| IBIS file was generated by Viper version: 2023.04.24
[IBIS Ver]   5.0
[Comment Char]   |_char
[File Name]   imxrt1180_c0_bga196_consmr.ibs
[File Rev]   1
[Date]   Thu Jan 23 17:55:28 2025
[Source]   NXP Viper 2023.04.24
[Notes]
[Disclaimer] IMPORTANT NOTICE
  This information is provided on an AS IS basis and without warranty.
  IN NO EVENT SHALL NXP BE LIABLE FOR INCIDENTAL OR CONSEQUENTIAL
  DAMAGES ARISING FROM USE OF THIS INFORMATION. THIS DISCLAIMER OF
  WARRANTY EXTENDS TO THE USER OF THE INFORMATION, AND TO THEIR CUSTOMERS
  OR USERS OF PRODUCTS  AND IS IN LIEU OF ALL WARRANTIES WHETHER EXPRESS,
  IMPLIED, OR STATUTORY, INCLUDING IMPLIED WARRANTIES OF MERCHANTABILITY
  OR FITNESS FOR PARTICULAR PURPOSE.
  NXP does not represent or warrant that the information furnished
  hereunder is free of infringement of any third party patents,
  copyrights, trade secrets, or other intellectual property rights.
  NXP does not represent or warrant that the information is free of
  defect, or that it meets any particular standard, requirements or need
  of the user of the infomation or their customers.
  NXP reserves the right to change the information in this file
  without notice.
   http://www.nxp.com
[Copyright]   (C) Copyright NXP 2004 - 2025, All Rights Reserved.
|   BGA196
[Component]   imxrt1180_bga196
[Manufacturer]   NXP
[Package]
| variable   typ   min   max
R_pkg   0.26256   0.042833   0.47223
L_pkg   3.535e-09   7.477e-10   7.758e-09
C_pkg   7.130e-13   4.458e-13   2.812e-12
[Pin] signal_name   model_name   R_pin   L_pin   C_pin
A1   VSS   GND   NA   NA   NA
A2   GPIO_EMC_B1_09   STGPIO   0.35642   4.603e-09 7.554e-13
A3   GPIO_AON_20   FSGPIO   0.21508   3.819e-09 5.831e-13
A4   GPIO_AON_19   FSGPIO   0.22197   4.065e-09 5.641e-13
A5   GPIO_AON_25   FSGPIO   0.3641   5.392e-09 5.514e-13
A6   GPIO_AON_24   FSGPIO   0.37702   4.913e-09 5.483e-13
A7   GPIO_AON_08   FSGPIO   0.37054   5.150e-09 5.122e-13
A8   GPIO_AON_12   FSGPIO   0.36547   5.045e-09 5.397e-13
A9   GPIO_AON_13   FSGPIO   0.39395   5.434e-09 5.821e-13
A10   GPIO_AON_01   FSGPIO   0.30629   5.038e-09 5.883e-13
A11   GPIO_AON_00   FSGPIO   0.29989   5.266e-09 6.848e-13
A12   GPIO_B2_07   STGPIO   0.47215   7.758e-09 9.398e-13
A13   GPIO_B2_08   STGPIO   0.47223   7.123e-09 9.633e-13
A14   VSS   GND   NA   NA   NA
B1   GPIO_EMC_B1_17   STGPIO   0.36515   4.326e-09 6.932e-13
B2   GPIO_EMC_B1_18   STGPIO   0.32419   3.726e-09 7.722e-13
B3   GPIO_AON_27   FSGPIO   0.26934   3.420e-09 5.231e-13
B4   GPIO_AON_26   FSGPIO   0.32404   4.795e-09 5.692e-13
B5   GPIO_AON_18   FSGPIO   0.24149   4.062e-09 5.595e-13
B6   GPIO_AON_23   FSGPIO   0.37852   5.044e-09 5.594e-13
B7   GPIO_AON_22   FSGPIO   0.39361   5.361e-09 5.709e-13
B8   GPIO_AON_15   FSGPIO   0.38558   5.824e-09 5.776e-13
B9   GPIO_AON_14   FSGPIO   0.40673   5.776e-09 6.039e-13
B10   GPIO_AON_11   FSGPIO   0.4088   6.162e-09 6.679e-13
B11   GPIO_AON_10   FSGPIO   0.40617   6.314e-09 6.924e-13
B12   GPIO_AON_09   FSGPIO   0.41769   6.788e-09 7.177e-13
B13   GPIO_B2_13   STGPIO   0.42759   6.730e-09 1.022e-12
B14   GPIO_B2_12   STGPIO   0.45182   7.389e-09 1.035e-12
C1   GPIO_EMC_B1_23   STGPIO   0.37543   4.204e-09 6.553e-13
C2   GPIO_EMC_B1_10   STGPIO   0.33639   3.642e-09 6.362e-13
C3   GPIO_EMC_B1_29   STGPIO   0.15709   2.341e-09 5.594e-13
C4   GPIO_AON_21   FSGPIO   0.10056   1.277e-09 6.902e-13
C5   GPIO_AON_17   FSGPIO   0.15303   1.931e-09 4.458e-13
C6   GPIO_AON_07   FSGPIO   0.15321   2.035e-09 4.695e-13
C7   GPIO_AON_06   FSGPIO   0.20767   2.944e-09 5.496e-13
C8   GPIO_AON_05   FSGPIO   0.26873   4.297e-09 6.302e-13
C9   GPIO_AON_02   FSGPIO   0.26227   4.486e-09 6.748e-13
C10   GPIO_B2_03   STGPIO   0.227   3.500e-09 9.260e-13
C11   GPIO_B2_05   STGPIO   0.28762   4.737e-09 9.986e-13
C12   GPIO_B2_00   STGPIO   0.32395   5.538e-09 1.004e-12
C13   GPIO_B2_10   STGPIO   0.41221   6.592e-09 8.958e-13
C14   GPIO_B2_11   STGPIO   0.44381   7.319e-09 9.732e-13
D1   GPIO_EMC_B1_15   STGPIO   0.36793   4.383e-09 6.235e-13
D2   GPIO_EMC_B1_20   STGPIO   0.34082   4.036e-09 6.104e-13
D3   GPIO_EMC_B1_11   STGPIO   0.34343   4.504e-09 6.504e-13
D4   VSS   GND   NA   NA   NA
D5   GPIO_EMC_B1_28   STGPIO   0.1112   1.432e-09 8.313e-13
D6   GPIO_AON_16   FSGPIO   0.09263   1.103e-09 5.826e-13
D7   NVCC_AON   POWER   NA   NA   NA
D8   GPIO_AON_03   FSGPIO   0.1963   3.001e-09 6.671e-13
D9   GPIO_B2_01   STGPIO   0.21713   2.881e-09 1.080e-12
D10   GPIO_B2_09   STGPIO   0.32026   5.525e-09 1.084e-12
D11   GPIO_B2_02   STGPIO   0.25143   3.934e-09 9.558e-13
D12   VSS   GND   NA   NA   NA
D13   USB1_DP   NC   0.2651   2.959e-09 6.312e-13
D14   USB1_DN   NC   0.25268   3.083e-09 6.395e-13
E1   GPIO_EMC_B1_05   STGPIO   0.23832   3.373e-09 6.272e-13
E2   GPIO_EMC_B1_16   STGPIO   0.31197   3.749e-09 6.419e-13
E3   GPIO_EMC_B1_13   STGPIO   0.1608   1.956e-09 6.369e-13
E4   GPIO_EMC_B1_19   STGPIO   0.098234  1.236e-09 7.015e-13
E5   GPIO_EMC_B1_12   STGPIO   0.098212  1.265e-09 6.870e-13
E6   GPIO_EMC_B1_03   STGPIO   0.13042   1.980e-09 8.047e-13
E7   GPIO_AON_04   FSGPIO   0.18605   2.492e-09 7.514e-13
E8   GPIO_B2_06   STGPIO   0.19268   2.582e-09 1.079e-12
E9   GPIO_B2_04   STGPIO   0.19249   2.700e-09 1.077e-12
E10   GPIO_SD_B1_03   STGPIO   0.24696   2.917e-09 9.185e-13
E11   VDD_USB_3P3   POWER   NA   NA   NA
E12   VDD_USB_1P8   POWER   NA   NA   NA
E13   GPIO_SD_B2_08   STGPIO   0.29716   3.541e-09 5.748e-13
E14   USB1_VBUS   POWER   0.18698   2.479e-09 6.560e-13
F1   GPIO_EMC_B1_31   STGPIO   0.34863   3.980e-09 5.917e-13
F2   GPIO_EMC_B1_30   STGPIO   0.31813   3.449e-09 5.603e-13
F3   GPIO_EMC_B1_08   STGPIO   0.17187   2.258e-09 6.398e-13
F4   GPIO_EMC_B1_14   STGPIO   0.15057   1.843e-09 6.464e-13
F5   GPIO_EMC_B1_01   STGPIO   0.11596   1.557e-09 7.297e-13
F6   NVCC_EMC1   POWER   NA   NA   NA
F7   VSS   GND   NA   NA   NA
F8   VSS   GND   NA   NA   NA
F9   VDD_SOC   POWER   NA   NA   NA
F10   GPIO_SD_B1_02   STGPIO   0.12357   1.900e-09 9.082e-13
F11   GPIO_SD_B2_03   STGPIO   0.21146   2.290e-09 6.433e-13
F12   GPIO_SD_B2_05   STGPIO   0.20101   2.322e-09 6.367e-13
F13   GPIO_SD_B2_11   STGPIO   0.29205   3.573e-09 5.872e-13
F14   GPIO_SD_B2_07   STGPIO   0.32121   4.153e-09 5.878e-13
G1   GPIO_EMC_B1_32   STGPIO   0.33057   3.828e-09 5.129e-13
G2   GPIO_EMC_B1_02   STGPIO   0.25413   3.884e-09 6.301e-13
G3   GPIO_EMC_B1_00   STGPIO   0.1527   1.898e-09 5.702e-13
G4   VSS   GND   NA   NA   NA
G5   GPIO_EMC_B1_27   STGPIO   0.19887   2.581e-09 7.781e-13
G6   NVCC_EMC1   POWER   NA   NA   NA
G7   VSS   GND   NA   NA   NA
G8   VDD_SOC   POWER   NA   NA   NA
G9   VDD_SOC   POWER   NA   NA   NA
G10   NVCC_SD2   POWER   NA   NA   NA
G11   VSS   GND   NA   NA   NA
G12   GPIO_SD_B2_04   STGPIO   0.20136   2.455e-09 5.936e-13
G13   GPIO_SD_B2_06   STGPIO   0.29033   3.676e-09 6.032e-13
G14   GPIO_SD_B2_09   STGPIO   0.31752   4.313e-09 5.550e-13
H1   GPIO_EMC_B1_33   STGPIO   0.34284   3.995e-09 5.590e-13
H2   GPIO_EMC_B1_35   STGPIO   0.31001   3.663e-09 5.512e-13
H3   GPIO_EMC_B1_34   STGPIO   0.31772   4.079e-09 5.714e-13
H4   GPIO_EMC_B1_06   STGPIO   0.16355   2.111e-09 7.119e-13
H5   GPIO_EMC_B1_04   STGPIO   0.1908   2.611e-09 7.576e-13
H6   GPIO_EMC_B1_21   STGPIO   0.18972   2.544e-09 7.609e-13
H7   VSS   GND   NA   NA   NA
H8   VDD_SOC   POWER   NA   NA   NA
H9   VDD_SOC   POWER   NA   NA   NA
H10   NVCC_SD2   POWER   NA   NA   NA
H11   GPIO_SD_B2_01   STGPIO   0.22799   3.317e-09 6.041e-13
H12   VDDA_ADC_3P3   POWER   NA   NA   NA
H13   GPIO_SD_B2_10   STGPIO   0.30632   3.978e-09 5.504e-13
H14   GPIO_SD_B2_02   STGPIO   0.33652   3.878e-09 5.752e-13
J1   GPIO_EMC_B1_37   STGPIO   0.32323   3.485e-09 5.526e-13
J2   GPIO_EMC_B1_36   STGPIO   0.37907   4.542e-09 6.302e-13
J3   GPIO_EMC_B1_24   STGPIO   0.15666   1.982e-09 5.863e-13
J4   GPIO_EMC_B1_22   STGPIO   0.17751   2.520e-09 6.260e-13
J5   GPIO_EMC_B1_07   STGPIO   0.10368   1.310e-09 6.824e-13
J6   GPIO_EMC_B1_25   STGPIO   0.18635   2.288e-09 8.252e-13
J7   GPIO_EMC_B1_26   STGPIO   0.2608   3.161e-09 8.827e-13
J8   GPIO_EMC_B2_12   STGPIO   0.19517   3.479e-09 8.111e-13
J9   GPIO_BBSM_05   NC   0.1742   2.674e-09 8.790e-13
J10   VDDA_1P8_IN   POWER   NA   NA   NA
J11   GPIO_SD_B2_00   STGPIO   0.2566   3.930e-09 6.694e-13
J12   DAC_OUT   NC   0.10066   1.340e-09 6.040e-13
J13   VDDA_ADC_1P8   POWER   NA   NA   NA
J14   ADC_VREFH   NC   0.17697   2.908e-09 6.279e-13
K1   GPIO_EMC_B1_39   STGPIO   0.33974   4.342e-09 5.830e-13
K2   GPIO_EMC_B1_38   STGPIO   0.35126   4.532e-09 6.394e-13
K3   DCDC_PSWITCH   NC   0.24821   2.705e-09 6.677e-13
K4   VSS   GND   NA   NA   NA
K5   DCDC_1P8   POWER   0.11971   1.732e-09 9.329e-13
K6   GPIO_EMC_B2_02   STGPIO   0.16558   2.154e-09 6.342e-13
K7   NVCC_EMC2   POWER   NA   NA   NA
K8   VSS   GND   NA   NA   NA
K9   VDD_BBSM_IN   POWER   NA   NA   NA
K10   VDD_AON_DIG   POWER   NA   NA   NA
K11   NVCC_GPIO_AD   POWER   NA   NA   NA
K12   VSS   GND   NA   NA   NA
K13   GPIO_AD_19   FSGPIO   0.19305   2.641e-09 6.018e-13
K14   GPIO_AD_31   FSGPIO   0.33197   4.295e-09 6.229e-13
L1   GPIO_EMC_B1_40   STGPIO   0.34095   4.119e-09 6.597e-13
L2   GPIO_EMC_B1_41   STGPIO   0.30369   3.628e-09 6.140e-13
L3   DCDC_SENSE   POWER   0.26018   3.078e-09 6.504e-13
L4   DCDC_IN_Q   POWER   0.12919   1.624e-09 7.804e-13
L5   GPIO_EMC_B2_00   STGPIO   0.16247   2.223e-09 6.129e-13
L6   GPIO_EMC_B2_01   STGPIO   0.094941  1.279e-09 6.311e-13
L7   GPIO_EMC_B2_11   STGPIO   0.16091   2.245e-09 6.729e-13
L8   GPIO_EMC_B2_07   STGPIO   0.16233   2.086e-09 6.342e-13
L9   VDD_BBSM_ANA   POWER   NA   NA   NA
L10   VDD_AON_ANA   POWER   NA   NA   NA
L11   GPIO_AD_15   FSGPIO   0.11573   1.752e-09 7.719e-13
L12   GPIO_AD_17   FSGPIO   0.27714   3.254e-09 7.574e-13
L13   GPIO_AD_18   FSGPIO   0.17013   2.631e-09 6.297e-13
L14   GPIO_AD_30   FSGPIO   0.32048   4.177e-09 6.164e-13
M1   DCDC_IN   POWER   NA   NA   NA
M2   DCDC_IN   POWER   NA   NA   NA
M3   DCDC_IN   POWER   NA   NA   NA
M4   DCDC_GND   GND   NA   NA   NA
M5   GPIO_EMC_B2_08   STGPIO   0.31954   3.205e-09 6.715e-13
M6   GPIO_EMC_B2_03   STGPIO   0.31024   3.351e-09 6.278e-13
M7   GPIO_EMC_B2_10   STGPIO   0.14582   1.718e-09 5.855e-13
M8   GPIO_EMC_B2_20   STGPIO   0.30924   3.774e-09 6.080e-13
M9   NVCC_BBSM   POWER   NA   NA   NA
M10   VDDA_1P0   POWER   NA   NA   NA
M11   GPIO_AD_14   FSGPIO   0.13042   2.291e-09 8.541e-13
M12   GPIO_AD_13   FSGPIO   0.12995   2.139e-09 6.989e-13
M13   GPIO_AD_12   FSGPIO   0.29034   3.434e-09 7.746e-13
M14   GPIO_AD_29   FSGPIO   0.24357   3.529e-09 6.917e-13
N1   DCDC_LP   POWER   NA   NA   NA
N2   DCDC_LP   POWER   NA   NA   NA
N3   DCDC_LP   POWER   NA   NA   NA
N4   DCDC_GND   GND   NA   NA   NA
N5   GPIO_EMC_B2_05   STGPIO   0.29445   3.095e-09 6.311e-13
N6   GPIO_EMC_B2_09   STGPIO   0.2938   3.454e-09 5.857e-13
N7   GPIO_EMC_B2_19   STGPIO   0.31237   3.127e-09 5.548e-13
N8   PMIC_ON_REQ   NC   0.28335   3.680e-09 5.528e-13
N9   TEST_MODE   NC   0.29046   3.631e-09 5.607e-13
N10   RTC_XTALI   NC   0.20653   2.835e-09 6.498e-13
N11   GPIO_BBSM_00   NC   0.37149   5.223e-09 6.873e-13
N12   CLK1_N   NC   0.32436   3.600e-09 8.673e-13
N13   XTALO   NC   0.34448   4.177e-09 8.140e-13
N14   GPIO_AD_16   FSGPIO   0.34349   4.680e-09 7.587e-13
P1   VSS   GND   NA   NA   NA
P2   DCDC_LP   POWER   NA   NA   NA
P3   DCDC_LP   POWER   NA   NA   NA
P4   DCDC_GND   GND   NA   NA   NA
P5   GPIO_EMC_B2_04   STGPIO   0.31706   3.733e-09 6.038e-13
P6   GPIO_EMC_B2_06   STGPIO   0.32474   3.906e-09 5.859e-13
P7   WAKEUP   NC   0.31367   4.177e-09 5.941e-13
P8   ONOFF   NC   0.31554   4.202e-09 5.713e-13
P9   POR_B   NC   0.32269   4.317e-09 5.737e-13
P10   RTC_XTALO   NC   0.21344   2.915e-09 6.504e-13
P11   VDD_AON_IN   POWER   NA   NA   NA
P12   CLK1_P   NC   0.33749   3.600e-09 8.878e-13
P13   XTALI   NC   0.33314   4.274e-09 7.732e-13
P14   VSS   GND   NA   NA   NA
[Pin Mapping]   pulldown_ref   pullup_ref
A1   VSS   NC
A2   VSS   NVCC_EMC1
A3   VSS   NVCC_AON
A4   VSS   NVCC_AON
A5   VSS   NVCC_AON
A6   VSS   NVCC_AON
A7   VSS   NVCC_AON
A8   VSS   NVCC_AON
A9   VSS   NVCC_AON
A10   VSS   NVCC_AON
A11   VSS   NVCC_AON
A12   VSS   NVCC_GPIO_AD
A13   VSS   NVCC_GPIO_AD
A14   VSS   NC
B1   VSS   NVCC_EMC1
B2   VSS   NVCC_EMC1
B3   VSS   NVCC_AON
B4   VSS   NVCC_AON
B5   VSS   NVCC_AON
B6   VSS   NVCC_AON
B7   VSS   NVCC_AON
B8   VSS   NVCC_AON
B9   VSS   NVCC_AON
B10   VSS   NVCC_AON
B11   VSS   NVCC_AON
B12   VSS   NVCC_AON
B13   VSS   NVCC_GPIO_AD
B14   VSS   NVCC_GPIO_AD
C1   VSS   NVCC_EMC1
C2   VSS   NVCC_EMC1
C3   VSS   NVCC_EMC1
C4   VSS   NVCC_AON
C5   VSS   NVCC_AON
C6   VSS   NVCC_AON
C7   VSS   NVCC_AON
C8   VSS   NVCC_AON
C9   VSS   NVCC_AON
C10   VSS   NVCC_GPIO_AD
C11   VSS   NVCC_GPIO_AD
C12   VSS   NVCC_GPIO_AD
C13   VSS   NVCC_GPIO_AD
C14   VSS   NVCC_GPIO_AD
D1   VSS   NVCC_EMC1
D2   VSS   NVCC_EMC1
D3   VSS   NVCC_EMC1
D4   VSS   NC
D5   VSS   NVCC_EMC1
D6   VSS   NVCC_AON
D7   NC   NVCC_AON
D8   VSS   NVCC_AON
D9   VSS   NVCC_GPIO_AD
D10   VSS   NVCC_GPIO_AD
D11   VSS   NVCC_GPIO_AD
D12   VSS   NC
D13   NC   NC
D14   NC   NC
E1   VSS   NVCC_EMC1
E2   VSS   NVCC_EMC1
E3   VSS   NVCC_EMC1
E4   VSS   NVCC_EMC1
E5   VSS   NVCC_EMC1
E6   VSS   NVCC_EMC1
E7   VSS   NVCC_AON
E8   VSS   NVCC_GPIO_AD
E9   VSS   NVCC_GPIO_AD
E10   VSS   NVCC_SD2
E11   NC   VDD_USB_3P3
E12   NC   VDD_USB_1P8
E13   VSS   NVCC_SD2
E14   NC   VDD_USB_3P3
F1   VSS   NVCC_EMC1
F2   VSS   NVCC_EMC1
F3   VSS   NVCC_EMC1
F4   VSS   NVCC_EMC1
F5   VSS   NVCC_EMC1
F6   NC   NVCC_EMC1
F7   VSS   NC
F8   VSS   NC
F9   NC   VDD_SOC
F10   VSS   NVCC_SD2
F11   VSS   NVCC_SD2
F12   VSS   NVCC_SD2
F13   VSS   NVCC_SD2
F14   VSS   NVCC_SD2
G1   VSS   NVCC_EMC1
G2   VSS   NVCC_EMC1
G3   VSS   NVCC_EMC1
G4   VSS   NC
G5   VSS   NVCC_EMC1
G6   NC   NVCC_EMC1
G7   VSS   NC
G8   NC   VDD_SOC
G9   NC   VDD_SOC
G10   NC   NVCC_SD2
G11   VSS   NC
G12   VSS   NVCC_SD2
G13   VSS   NVCC_SD2
G14   VSS   NVCC_SD2
H1   VSS   NVCC_EMC1
H2   VSS   NVCC_EMC1
H3   VSS   NVCC_EMC1
H4   VSS   NVCC_EMC1
H5   VSS   NVCC_EMC1
H6   VSS   NVCC_EMC1
H7   VSS   NC
H8   NC   VDD_SOC
H9   NC   VDD_SOC
H10   NC   NVCC_SD2
H11   VSS   NVCC_SD2
H12   NC   VDDA_ADC_3P3
H13   VSS   NVCC_SD2
H14   VSS   NVCC_SD2
J1   VSS   NVCC_EMC1
J2   VSS   NVCC_EMC1
J3   VSS   NVCC_EMC1
J4   VSS   NVCC_EMC1
J5   VSS   NVCC_EMC1
J6   VSS   NVCC_EMC1
J7   VSS   NVCC_EMC1
J8   VSS   NVCC_EMC2
J9   NC   NC
J10   NC   VDDA_1P8_IN
J11   VSS   NVCC_SD2
J12   NC   NC
J13   NC   VDDA_ADC_1P8
J14   NC   NC
K1   VSS   NVCC_EMC1
K2   VSS   NVCC_EMC1
K3   NC   NC
K4   VSS   NC
K5   NC   DCDC_1P8
K6   VSS   NVCC_EMC2
K7   NC   NVCC_EMC2
K8   VSS   NC
K9   NC   VDD_BBSM_IN
K10   NC   VDD_AON_DIG
K11   NC   NVCC_GPIO_AD
K12   VSS   NC
K13   VSS   NVCC_GPIO_AD
K14   VSS   NVCC_GPIO_AD
L1   VSS   NVCC_EMC1
L2   VSS   NVCC_EMC1
L3   NC   DCDC_SENSE
L4   NC   DCDC_IN_Q
L5   VSS   NVCC_EMC2
L6   VSS   NVCC_EMC2
L7   VSS   NVCC_EMC2
L8   VSS   NVCC_EMC2
L9   NC   VDD_BBSM_ANA
L10   NC   VDD_AON_ANA
L11   VSS   NVCC_GPIO_AD
L12   VSS   NVCC_GPIO_AD
L13   VSS   NVCC_GPIO_AD
L14   VSS   NVCC_GPIO_AD
M1   NC   DCDC_IN
M2   NC   DCDC_IN
M3   NC   DCDC_IN
M4   DCDC_GND   NC
M5   VSS   NVCC_EMC2
M6   VSS   NVCC_EMC2
M7   VSS   NVCC_EMC2
M8   VSS   NVCC_EMC2
M9   NC   NVCC_BBSM
M10   NC   VDDA_1P0
M11   VSS   NVCC_GPIO_AD
M12   VSS   NVCC_GPIO_AD
M13   VSS   NVCC_GPIO_AD
M14   VSS   NVCC_GPIO_AD
N1   NC   DCDC_LP
N2   NC   DCDC_LP
N3   NC   DCDC_LP
N4   DCDC_GND   NC
N5   VSS   NVCC_EMC2
N6   VSS   NVCC_EMC2
N7   VSS   NVCC_EMC2
N8   NC   NC
N9   NC   NC
N10   NC   NC
N11   NC   NC
N12   NC   NC
N13   NC   NC
N14   VSS   NVCC_GPIO_AD
P1   VSS   NC
P2   NC   DCDC_LP
P3   NC   DCDC_LP
P4   DCDC_GND   NC
P5   VSS   NVCC_EMC2
P6   VSS   NVCC_EMC2
P7   NC   NC
P8   NC   NC
P9   NC   NC
P10   NC   NC
P11   NC   VDD_AON_IN
P12   NC   NC
P13   NC   NC
P14   VSS   NC
|*   Model Selector   *
[Model Selector] STGPIO
BDPROGSCARUDQP_SDMMC_3V3SF_00_SD   PSW=0 High Drive, 1V8 SD
BDPROGSCARUDQP_SDMMC_3V3SF_01_SD   PSW=0 Low Drive,  1V8 SD
BDPROGSCARUDQP_SDMMC_3V3SF_00_MMC   PSW=0 High Drive, 1V8 MMC
BDPROGSCARUDQP_SDMMC_3V3SF_01_MMC   PSW=0 Low Drive,  1V8 MMC
BDPROGSCARUDQP_SDMMC_3V3SF_10   PSW=1 High Drive, 3V3 +/- 10%, SD & 3V3 MMC
BDPROGSCARUDQP_SDMMC_3V3SF_11   PSW=1 Low Drive,  3V3 +/- 10%, SD & 3V3 MMC
BDPROGSCARUDQP_SDMMC_3V3SF_10_5pct  PSW=1 High Drive, 3V3 +/- 5%, SD & 3V3 MMC
BDPROGSCARUDQP_SDMMC_3V3SF_11_5pct  PSW=1 Low Drive,  3V3 +/- 5%, SD & 3V3 MMC
BDPROGSCARUDQP_SDMMC_3V3SF_11_2v7   PSW=1 Low Drive,  2V7 SD & 2V7 MMC
BDPROGSCARUDQP_SDMMC_3V3SF_10_2v7   PSW=1 High Drive, 2V7 SD & 2V7 MMC
[Model Selector] FSGPIO
io_crnrobe1dse0sre0   Normal range in cont mode, 5mA drive strength, without slew rate
io_crnrobe1dse0sre1   Normal range in cont mode, 5mA drive strength, with slew rate
io_crnrobe1dse1sre0   Normal range in cont mode, 10mA drive strength, without slew rate
io_crnrobe1dse1sre1   Normal range in cont mode, 10mA drive strength, with slew rate
io_crdrobe1dse0sre0   Derated range in cont mode, 5mA drive strength, without slew rate
io_crdrobe1dse0sre1   Derated range in cont mode, 5mA drive strength, with slew rate
io_crdrobe1dse1sre0   Derated range in cont mode, 10mA drive strength, without slew rate
io_crdrobe1dse1sre1   Derated range in cont mode, 10mA drive strength, with slew rate
io_crdr2obe1dse0sre0   Derated2 range in cont mode, 5mA drive strength, without slew rate
io_crdr2obe1dse0sre1   Derated2 range in cont mode, 5mA drive strength, with slew rate
io_crdr2obe1dse1sre0   Derated2 range in cont mode, 10mA drive strength, without slew rate
io_crdr2obe1dse1sre1   Derated2 range in cont mode, 10mA drive strength, with slew rate
io_hrobe1dse0sre0   high range mode, 5mA drive strength, without slew rate
io_hrobe1dse0sre1   high range mode, 5mA drive strength, with slew rate
io_hrobe1dse1sre0   high range mode, 10mA drive strength, without slew rate
io_hrobe1dse1sre1   high range mode, 10mA drive strength, with slew rate
io_lrobe1dse0sre0   low range mode, 5mA drive strength, without slew rate
io_lrobe1dse0sre1   low range mode, 5mA drive strength, with slew rate
io_lrobe1dse1sre0   low range mode, 10mA drive strength, without slew rate
io_lrobe1dse1sre1   low range mode, 10mA drive strength, with slew rate
io_crnrobe1dse0sre0_5pct   Narrow range in cont mode, 5mA drive strength, without slew rate
io_crnrobe1dse0sre1_5pct   Narrow range in cont mode, 5mA drive strength, with slew rate
io_crnrobe1dse1sre0_5pct   Narrow range in cont mode, 10mA drive strength, without slew rate
io_crnrobe1dse1sre1_5pct   Narrow range in cont mode, 10mA drive strength, with slew rate
io_hrobe1dse0sre0_5pct   Narrow range in high range mode, 5mA drive strength, without slew rate
io_hrobe1dse0sre1_5pct   Narrow range in high range mode, 5mA drive strength, with slew rate
io_hrobe1dse1sre0_5pct   Narrow range in high range mode, 10mA drive strength, without slew rate
io_hrobe1dse1sre1_5pct   Narrow range in high range mode, 10mA drive strength, with slew rate
|End  [Component] imxrt1180_bga196
| Models and submodels in the file (38): BDPROGSCARUDQP_SDMMC_3V3SF_00_MMC (I/O), BDPROGSCARUDQP_SDMMC_3V3SF_00_SD (I/O), BDPROGSCARUDQP_SDMMC_3V3SF_01_MMC (I/O), BDPROGSCARUDQP_SDMMC_3V3SF_01_SD (I/O), BDPROGSCARUDQP_SDMMC_3V3SF_10 (I/O), BDPROGSCARUDQP_SDMMC_3V3SF_11 (I/O), BDPROGSCARUDQP_SDMMC_3V3SF_10_2v7 (I/O), BDPROGSCARUDQP_SDMMC_3V3SF_11_2v7 (I/O), BDPROGSCARUDQP_SDMMC_3V3SF_10_5pct (I/O), BDPROGSCARUDQP_SDMMC_3V3SF_11_5pct (I/O), io_crnrobe1dse0sre0 (I/O), io_crnrobe1dse0sre1 (I/O), io_crnrobe1dse1sre0 (I/O), io_crnrobe1dse1sre1 (I/O), io_crdrobe1dse0sre0 (I/O), io_crdrobe1dse0sre1 (I/O), io_crdrobe1dse1sre0 (I/O), io_crdrobe1dse1sre1 (I/O), io_crdr2obe1dse0sre0 (I/O), io_crdr2obe1dse0sre1 (I/O), io_crdr2obe1dse1sre0 (I/O), io_crdr2obe1dse1sre1 (I/O), io_hrobe1dse0sre0 (I/O), io_hrobe1dse0sre1 (I/O), io_hrobe1dse1sre0 (I/O), io_hrobe1dse1sre1 (I/O), io_lrobe1dse0sre0 (I/O), io_lrobe1dse0sre1 (I/O), io_lrobe1dse1sre0 (I/O), io_lrobe1dse1sre1 (I/O), io_crnrobe1dse0sre0_5pct (I/O), io_crnrobe1dse0sre1_5pct (I/O), io_crnrobe1dse1sre0_5pct (I/O), io_crnrobe1dse1sre1_5pct (I/O), io_hrobe1dse0sre0_5pct (I/O), io_hrobe1dse0sre1_5pct (I/O), io_hrobe1dse1sre0_5pct (I/O), io_hrobe1dse1sre1_5pct (I/O)
